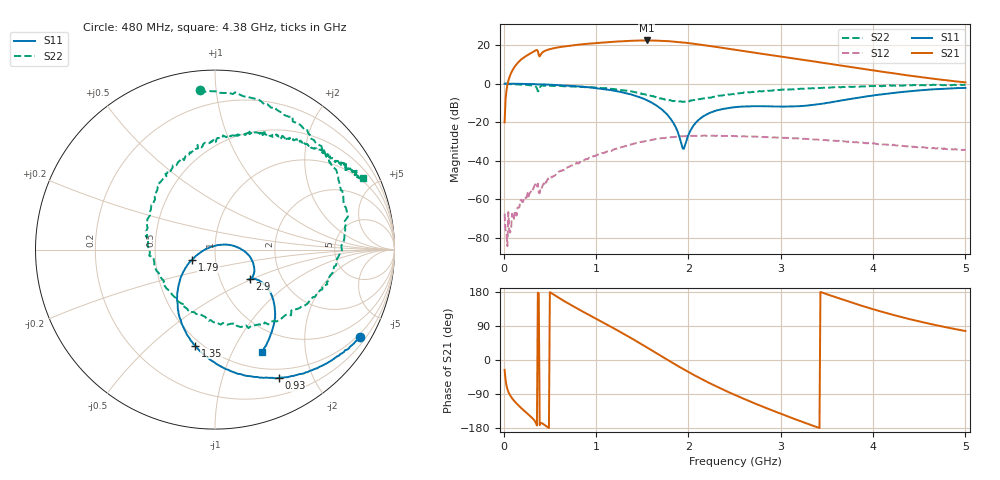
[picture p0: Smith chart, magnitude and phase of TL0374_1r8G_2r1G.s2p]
! Created Fri Jul 02 06:36:55 2021
# hz S ri R 50
! 2 Port Network Data from SP1.SP block
! freq  reS11  imS11  reS21  imS21  reS12  imS12  reS22  imS22
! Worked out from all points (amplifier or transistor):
!   500 points, 10 MHz to 5 GHz, reference 50 ohm
!   highest |S21| = 22.4 dB at 1.55 GHz (marker M1)
!   |S21| within 3 dB of that: 671.6 MHz to 2.249 GHz (1.577 GHz wide, 108 % of centre)
!   unconditionally stable (mu >= 1): 262.8 MHz to 474.2 MHz; 795.2 MHz to 851.2 MHz; 865.1 MHz to end of sweep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
!   at 840 MHz: K = 1.02, MAG = 29.5 dB, |S12| = -40.2 dB
!   at 2.51 GHz: K = 1.17, MAG = 19.9 dB, |S12| = -27.3 dB
!   at 5 GHz: K = 1.94, MAG = 12.0 dB, |S12| = -34.6 dB
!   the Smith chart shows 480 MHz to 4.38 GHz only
!   S11 on the Smith chart (normalised r, x): 480 MHz: 0.40, -3.55; 930 MHz: 0.39, -1.54; 1.35 GHz: 0.46, -0.70; 1.79 GHz: 0.77, -0.09; 2.9 GHz: 1.38, -0.49; 4.38 GHz: 0.69, -1.31
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1e7  0.9949 -0.0123  0.0886 -0.0431  0.000413 6.12e-05  0.3095 -0.9572
2.3e8  0.9533 -0.2525  -3.568 -3.49  -0.000717 0.000898  -0.671 0.6401
3.5e8  0.8877 -0.3761  -7.173 -1.705  -0.000889 0.0024  -0.2283 0.7906
4e8  0.863 -0.4126  -5.461 -1.283  -0.00101 0.00171  -0.3697 0.7686
4.8e8  0.8077 -0.4877  -7.602 -0.2745  -0.00156 0.00304  -0.0859 0.891
6.4e8  0.67 -0.6027  -8.443 3.457  -0.00151 0.00548  0.2744 0.8098
8.5e8  0.4489 -0.6999  -6.585 8.182  0.000568 0.00978  0.5762 0.585
9.3e8  0.3556 -0.7146  -5.15 9.652  0.00239 0.0116  0.6421 0.4854
1.16e9  0.0803 -0.6737  0.4348 12.08  0.00962 0.0154  0.7256 0.1157
1.35e9  -0.1103 -0.5347  6.026 11.35  0.02 0.0153  0.6259 -0.1931
1.55e9  -0.2081 -0.3071  11.05 7.259  0.0319 0.00774  0.3123 -0.4008
1.68e9  -0.1908 -0.1546  12.64 3.218  0.0373 -0.00175  0.0674 -0.4188
1.79e9  -0.1275 -0.0554  12.63 -0.4133  0.0383 -0.0117  -0.1159 -0.3484
1.96e9  0.00521 0.0231  10.41 -5.101  0.0336 -0.0265  -0.314 -0.13
2.12e9  0.1179 0.0162  7.017 -7.614  0.0241 -0.037  -0.3827 0.1052
2.3e9  0.1952 -0.0404  3.173 -8.385  0.00995 -0.0428  -0.3194 0.3499
2.51e9  0.2198 -0.1105  -0.3795 -7.528  -0.00522 -0.0428  -0.1628 0.5231
2.9e9  0.1948 -0.1651  -3.672 -4.053  -0.0272 -0.0301  0.1614 0.6409
3.34e9  0.2248 -0.1644  -3.8 -0.4929  -0.0351 -0.00795  0.4548 0.6161
4.17e9  0.3176 -0.4539  -1.024 1.627  -0.0184 0.0182  0.772 0.4373
4.38e9  0.2604 -0.5718  -0.5217 1.544  -0.0128 0.0196  0.8226 0.397
5e9  -0.0833 -0.7699  0.2519 1.049  -0.00243 0.0185  0.8344 0.3716
